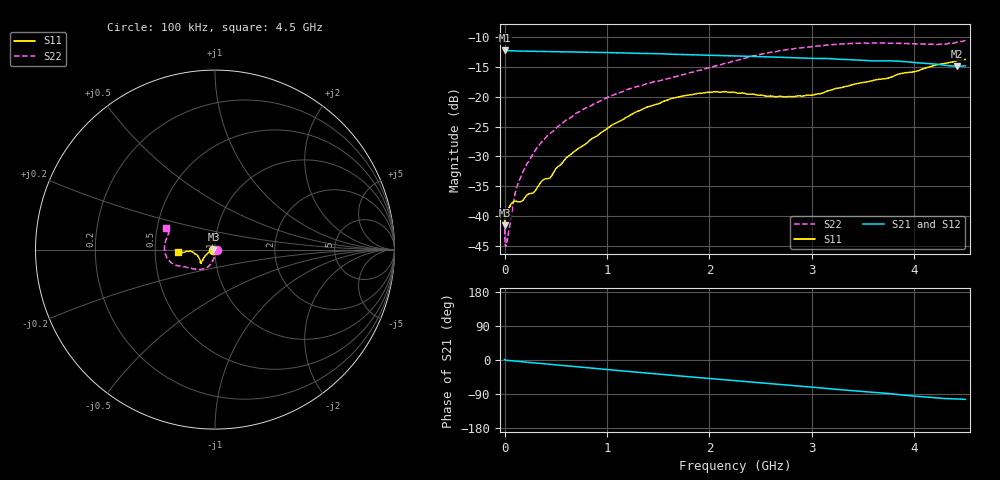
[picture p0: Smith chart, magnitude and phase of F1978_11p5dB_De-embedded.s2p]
! Integrated Device Technology
! Corporate Headquarters
! 6024 Silver Creek Valley Road
! San Jose, CA 95138  USA
! Phone:  1-408-284-8200
! Toll Free:  1-800-223-1366
! Webpage:  http://www.idt.com/
! Timing and RF Division
! 515 Groton Road, Suite 102
! Westford, MA 01886-6024
! Device:  F1978
! Description: 6-bit, 75 ohm, 0.5 dB Digital Step Attenuator
! Frequency:  5.0 MHz -  3.00 GHz
! Package:  4x4 mm QFN Plastic Package: 20 pin
! Ports:  2 RF, 11 DC
!  Pin  1  = D5 (16 dB)
!  Pin  2  = RF1  =  Port 1
!  Pin  3  = Serial Data In (DATA)
!  Pin  4  = Serial Clock (CLK)
!  Pin  5  = Serial Latch Enable (LE)
!  Pin  6  = VDD
!  Pin  7  = NC
!  Pin  8  = NC
!  Pin  9  = NC
!  Pin 10  = GND
!  Pin 11  = GND
!  Pin 12  = NC
!  Pin 13  = VMODE
!  Pin 14  = RF2  =  Port 2
!  Pin 15  = D4 (8 dB)
!  Pin 16  = D3 (4 dB)
!  Pin 17  = D2 (2 dB)
!  Pin 18  = NC
!  Pin 19  = D1 (1 dB)
!  Pin 20  = D0 (0.5 dB)
! State:  23
! Atten State:  11.5 dB
! Voltage:  +3.30 Volts
! Current:  0.565 mA
! Data:  The device was measured on a F1975 evaluation board which has
!  individual transmission lines to the RF pins.  Data was collected
!  using a calibrated network analyzer.  The evaluation board was
!  de-embedded using Automatic Fixture Removal (AFR).
!  The reference plane is the edge of the package pin.
! Misc:
!  Action Tracker AT0416
! Date Measured:  2018-02-08
! Date:  2018-03-26  MJV
! Note:
!  Integrated Device Technology supplies this data as a sample of measured
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# GHz S dB R 75
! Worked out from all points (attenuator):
!   291 points, 100 kHz to 4.5 GHz, reference 75 ohm
!   highest |S21| = -12.20 dB at 100 kHz (marker M1); lowest = -14.9 dB at 4.42 GHz (marker M2)
!   lowest |S11| = -41.5 dB at 100 kHz (marker M3), VSWR 1.02, Z = 73.8 - j0.0137 ohm
!   |S11| at or under -10 dB: start of sweep to end of sweep
!   |S22| runs from -45.0 to -10.6 dB; largest |S21 - S12| = 0.00019
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0.0001  -41.53 -179.4  -12.20 1.2  -12.20 1.2  -40.74 -1.6
0.001  -40.82 -176.7  -12.23 1.0  -12.23 1.0  -42.86 -10.5
0.003  -40.30 -176.6  -12.25 0.7  -12.25 0.7  -44.06 -15.3
0.006  -40.21 -176.0  -12.26 0.2  -12.26 0.2  -44.86 -23.7
0.013  -39.76 -174.9  -12.28 -0.6  -12.28 -0.5  -45.02 -40.3
0.1  -37.43 -167.0  -12.33 -2.9  -12.33 -2.9  -36.39 -92.6
0.16  -37.53 -166.1  -12.36 -4.4  -12.36 -4.4  -33.36 -91.6
0.22  -36.42 -167.3  -12.38 -5.9  -12.37 -5.9  -31.18 -92.6
0.28  -36.12 -165.6  -12.39 -7.4  -12.39 -7.4  -29.51 -95.8
0.36  -34.16 -165.9  -12.42 -9.4  -12.42 -9.4  -27.59 -96.1
0.42  -33.70 -162.2  -12.44 -10.9  -12.43 -10.9  -26.50 -96.8
0.6  -30.26 -161.7  -12.49 -15.3  -12.48 -15.3  -23.91 -100.8
0.76  -28.26 -155.6  -12.53 -19.2  -12.53 -19.2  -22.20 -104.6
1.06  -24.63 -148.8  -12.63 -26.5  -12.62 -26.5  -19.72 -111.9
1.52  -21.06 -139.6  -12.80 -37.5  -12.80 -37.5  -17.30 -126.1
1.88  -19.46 -136.3  -13.00 -46.0  -13.00 -46.0  -15.65 -139.8
2.26  -19.32 -138.3  -13.17 -54.7  -13.17 -54.7  -13.93 -151.6
2.64  -19.99 -148.3  -13.36 -63.6  -13.36 -63.5  -12.47 -159.2
3.02  -19.67 -163.5  -13.57 -72.1  -13.57 -72.1  -11.59 -166.8
3.76  -16.81 -176.0  -13.99 -88.7  -13.99 -88.7  -11.02 174.3
4.42  -13.90 -174.4  -14.89 -102.8  -14.89 -102.8  -10.84 157.7
4.5  -13.76 -176.3  -14.83 -104.0  -14.82 -104.0  -10.58 156.4
